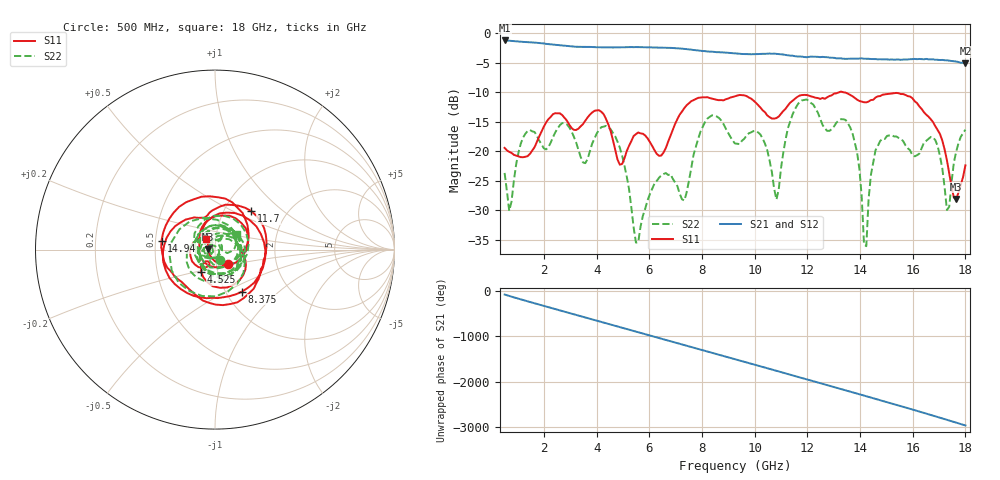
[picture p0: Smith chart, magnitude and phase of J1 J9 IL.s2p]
!Agilent Technologies,N5230A,MY45001360,A.07.50.67
!Agilent N5230A: A.07.50.67
!Date: Friday, April 12, 2024 22:07:12
!Correction: S11(Full 2 Port(1,2))
!S21(Full 2 Port(1,2))
!S12(Full 2 Port(1,2))
!S22(Full 2 Port(1,2))
!S2P File: Measurements: S11, S21, S12, S22:
# Hz S  dB  R 50
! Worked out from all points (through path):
!   201 points, 500 MHz to 18 GHz, reference 50 ohm
!   highest |S21| = -1.26 dB at 500 MHz (marker M1); lowest = -5.1 dB at 18 GHz (marker M2)
!   group delay of S21, straight-line fit = 456 ps
!   lowest |S11| = -28.1 dB at 17.65 GHz (marker M3), VSWR 1.08, Z = 46.2 + j0.246 ohm
!   |S11| at or under -10 dB: start of sweep to 13.22 GHz; 13.34 GHz to end of sweep
!   |S22| runs from -36.1 to -11.3 dB; largest |S21 - S12| = 0.0065
!   S11 on the Smith chart (normalised r, x): 500 MHz: 1.14, -0.18; 4.525 GHz: 0.83, -0.22; 8.375 GHz: 1.19, -0.60; 11.7 GHz: 1.34, +0.63; 14.94 GHz: 0.54, +0.06; 18 GHz: 0.90, +0.10
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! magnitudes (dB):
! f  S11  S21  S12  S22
! 500 MHz  -19.5  -1.3  -1.3  -23.7
! 2.688 GHz  -13.9  -2.1  -2.1  -15.3
! 3.475 GHz  -15.4  -2.3  -2.3  -21.9
! 4.525 GHz  -16.6  -2.4  -2.4  -16.3
! 5.487 GHz  -17.1  -2.4  -2.4  -35.5
! 6.362 GHz  -20.8  -2.5  -2.5  -24.5
! 7.325 GHz  -12.7  -2.7  -2.7  -28.4
! 8.375 GHz  -11.1  -3.2  -3.2  -14.0
! 9.25 GHz  -10.7  -3.5  -3.5  -18.7
! 10.21 GHz  -12.6  -3.5  -3.5  -17.2
! 10.82 GHz  -14.4  -3.5  -3.5  -28.2
! 11.7 GHz  -10.6  -4.0  -4.0  -11.7
! 12.22 GHz  -10.8  -4.0  -4.0  -12.1
! 13.71 GHz  -10.7  -4.3  -4.4  -17.0
! 14.24 GHz  -11.8  -4.4  -4.3  -36.1
! 14.41 GHz  -11.4  -4.4  -4.4  -24.0
! 14.94 GHz  -10.4  -4.5  -4.5  -18.0
! 15.11 GHz  -10.3  -4.5  -4.5  -17.4
! 16.77 GHz  -15.1  -4.5  -4.5  -17.7
! 17.3 GHz  -21.6  -4.6  -4.6  -30.0
! 17.65 GHz  -28.1  -4.8  -4.9  -20.1
! 18 GHz  -22.4  -5.1  -5.1  -16.4
